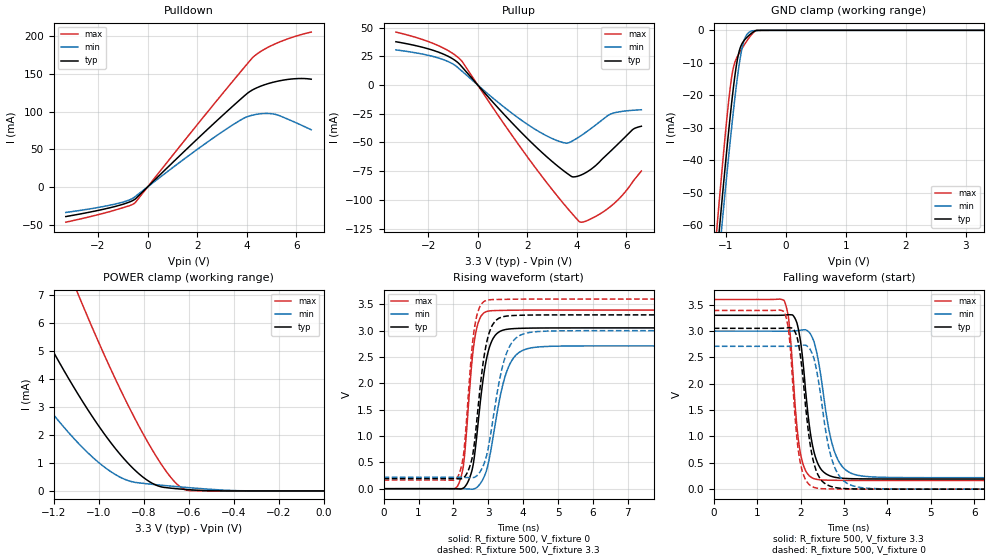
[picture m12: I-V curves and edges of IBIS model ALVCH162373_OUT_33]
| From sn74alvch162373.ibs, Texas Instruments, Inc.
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[Model]   ALVCH162373_OUT_33
Model_type  3-state
Enable   Active-Low
Vref =   0
Rref =   500
Cref =   50p
Vmeas =   1.5
| variable   typ   min   max
C_comp   6.78pF   5.76pF   8.31pF
| C_pullup   4.90pF   3.73pF   7.38pF
| C_pulldown   4.25pF   3.48pF   5.75pF
| C_tri-state   6.78pF   5.76pF   8.31pF
[Temperature Range]   40   100   -40
| Ambient temperature   25   85   -40
[Voltage range]   3.3   3   3.6
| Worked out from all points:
|   slope of the pulldown table from 0 to 0.495 V, typ, clamps not added: 31 ohm
|   slope of the pullup table from 0 to 0.495 V, typ, clamps not added: 40.8 ohm
|   GND clamp passes 1 mA (typ) near -0.58 V on its own axis
|   POWER clamp passes 1 mA (typ) near -0.87 V on its own axis
|   rising waveform, R_fixture 500, V_fixture 0: 20-80 % time 341ps typ, 481ps min, 256ps max; typ from 0 V to 3.05 V
|   falling waveform, R_fixture 500, V_fixture 3.3: 20-80 % time 260ps typ, 349ps min, 200ps max; typ from 3.3 V to 0.192 V
|   rising waveform, R_fixture 500, V_fixture 3.3: 20-80 % time 331ps typ, 460ps min, 252ps max; typ from 0.192 V to 3.3 V
|   falling waveform, R_fixture 500, V_fixture 0: 20-80 % time 264ps typ, 341ps min, 199ps max; typ from 3.05 V to 0 V
[GND Clamp]
| ALVCH162373_OUT_33
|   Voltage   I(typ)   I(min)   I(max)
-3.3V     -545.2mA   -539mA     -555.7mA
-1.16V    -72.15mA   -79.11mA   -63.54mA
-1.14V    -68.04mA   -75.1mA    -59.25mA
-1.1V     -59.88mA   -67.15mA   -50.77mA
-1.065V   -52.84mA   -60.28mA   -43.49mA
-920mV    -25.39mA   -33.03mA   -16.8mA
-870mV    -17.2mA    -24.4mA    -11.24mA
-815mV    -9.903mA   -15.76mA   -8.37mA
-710mV    -3.518mA   -4.058mA   -5.017mA
-585mV    -1.104mA   -317.1uA   -1.646mA
-465mV    -12.45uA   -47.91uA   -8.152uA
3.3V      114.4pA    941.2nA    51.31pA
[POWER Clamp]
| ALVCH162373_OUT_33
|   Voltage   I(typ)   I(min)   I(max)
-3.3V     45.5mA     34.01mA    62.51mA
-1.565V   10.81mA    6.981mA    17.27mA
-1.335V   7.004mA    4.173mA    12.09mA
-1.205V   5.038mA    2.778mA    9.335mA
-1.09V    3.449mA    1.71mA     7.028mA
-955mV    1.83mA     742.3uA    4.523mA
-835mV    718.9uA    302.8uA    2.539mA
-745mV    209.6uA    223.6uA    1.256mA
-690mV    109.3uA    182uA      600.5uA
-640mV    70.19uA    146.2uA    164.5uA
-570mV    29.05uA    98.95uA    5.202uA
-48.03fV  114.4pA    365.2pA    62.68pA
[Pulldown]
| ALVCH162373_OUT_33
|   Voltage   I(typ)   I(min)   I(max)
-3.3V     -39.36mA   -33.92mA   -46.84mA
-1.35V    -26.28mA   -23.06mA   -31.1mA
-795mV    -20.8mA    -18mA      -25.61mA
-510mV    -16.35mA   -13.06mA   -21.09mA
2.41V     76.27mA    59.51mA    99.29mA
3.47V     108.3mA    83.2mA     141.8mA
4.065V    125.4mA    93.8mA     165.3mA
4.25V     129.2mA    95.52mA    172.3mA
4.45V     132.4mA    96.76mA    177.5mA
5.14V     139.7mA    96.49mA    190mA
5.93V     143.7mA    86.07mA    199.8mA
6.6V      143.1mA    75.95mA    205.7mA
[Pullup]
| ALVCH162373_OUT_33
|   Voltage   I(typ)   I(min)   I(max)
-3.3V     37.7mA     30.59mA    46.11mA
-1.59V    28.69mA    23.58mA    34.31mA
-685mV    16.99mA    12.99mA    21.85mA
1.19V     -28.54mA   -21.41mA   -37.91mA
2.595V    -58.82mA   -42.14mA   -79.72mA
3.56V     -76.23mA   -50.65mA   -105.8mA
3.82V     -79.94mA   -48.68mA   -112.4mA
4.105V    -78.91mA   -44.96mA   -119.1mA
4.65V     -72.06mA   -36.57mA   -115.6mA
5.375V    -57.28mA   -25.16mA   -105.5mA
6.25V     -38.8mA    -22.01mA   -84.28mA
6.6V      -35.88mA   -21.54mA   -74.89mA
[Ramp]
| ALVCH162373_OUT_33
| variable   typ   min   max
dV/dt_r   1.84/3.48E-10   1.63/4.90E-10   2.04/2.64E-10
dV/dt_f   1.87/2.64E-10   1.69/3.58E-10   2.07/2.11E-10
R_load = 500
[Rising Waveform]
| ALVCH162373_OUT_33
R_fixture =   500
C_fixture =   0
L_fixture =   0
V_fixture =   0
V_fixture_min = 0
V_fixture_max = 0
|   Time   V(typ)   V(min)   V(max)
0s        350.5pV    1.172nV    255.3pV
2.12ns    -3.076mV   812uV      51.85mV
2.295ns   16.31mV    -1.798mV   482.8mV
2.52ns    316.9mV    -8.823mV   2.332V
2.62ns    709.3mV    3.587mV    2.884V
2.835ns   1.995V     164.5mV    3.31V
2.995ns   2.596V     465.5mV    3.371V
3.55ns    3.027V     2.262V     3.386V
4.28ns    3.049V     2.679V     3.391V
24.99ns   3.053V     2.712V     3.391V
[Falling Waveform]
| ALVCH162373_OUT_33
R_fixture =   500
C_fixture =   0
L_fixture =   0
V_fixture =   3.3
V_fixture_min = 3
V_fixture_max = 3.6
|   Time   V(typ)   V(min)   V(max)
0s        3.3V       3V         3.6V
1.62ns    3.303V     2.998V     3.582V
1.735ns   3.311V     2.998V     3.155V
1.9ns     3.189V     3.005V     1.332V
1.995ns   2.824V     3.017V     687.2mV
2.215ns   1.127V     2.961V     242.5mV
2.385ns   509mV      2.541V     183.7mV
2.795ns   224.9mV    680.4mV    168.4mV
3.45ns    195.3mV    245.1mV    165.3mV
24.99ns   192.3mV    217.1mV    164.5mV
[Rising Waveform]
| ALVCH162373_OUT_33
R_fixture =   500
C_fixture =   0
L_fixture =   0
V_fixture =   3.3
V_fixture_min = 3
V_fixture_max = 3.6
|   Time   V(typ)   V(min)   V(max)
0s        192.3mV    217.1mV    164.5mV
2.115ns   189mV      217.3mV    213.1mV
2.295ns   210.2mV    214.4mV    675.1mV
2.515ns   523.5mV    207.9mV    2.537V
2.615ns   942.1mV    220.7mV    3.1V
2.83ns    2.281V     396.8mV    3.524V
2.985ns   2.866V     729mV      3.582V
3.51ns    3.276V     2.549V     3.595V
4.2ns     3.296V     2.968V     3.599V
24.99ns   3.3V       3V         3.6V
[Falling Waveform]
| ALVCH162373_OUT_33
R_fixture =   500
C_fixture =   0
L_fixture =   0
V_fixture =   0
V_fixture_min = 0
V_fixture_max = 0
|   Time   V(typ)   V(min)   V(max)
0s        3.053V     2.712V     3.391V
1.62ns    3.056V     2.711V     3.372V
1.73ns    3.063V     2.711V     2.97V
1.895ns   2.943V     2.717V     1.147V
1.99ns    2.561V     2.728V     517mV
2.205ns   935.2mV    2.671V     82.35mV
2.385ns   299mV      2.184V     18.24mV
2.775ns   35.02mV    434.5mV    3.551mV
3.42ns    2.728mV    27.19mV    638.2uV
24.99ns   -7.069nV   2.343nV    323.1pV
